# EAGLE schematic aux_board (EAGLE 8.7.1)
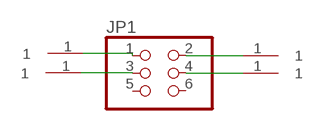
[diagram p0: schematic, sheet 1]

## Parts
JP1  PIN_HEADER_SMD_2X3  [2X03SMD]
U$2  FABRIC_PIN  [FABRIC_PIN]
U$3  FABRIC_PIN  [FABRIC_PIN]
U$4  FABRIC_PIN  [FABRIC_PIN]
U$5  FABRIC_PIN  [FABRIC_PIN]

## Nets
N$1: JP1.1 U$3.1
N$2: JP1.3 U$2.1
N$3: JP1.2 U$4.1
N$4: JP1.4 U$5.1
Unconnected: JP1.5 JP1.6

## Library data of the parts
JP1 = fab:PIN_HEADER_SMD_2X3: PIN HEADER
U$2-U$5 = fab:FABRIC_PIN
